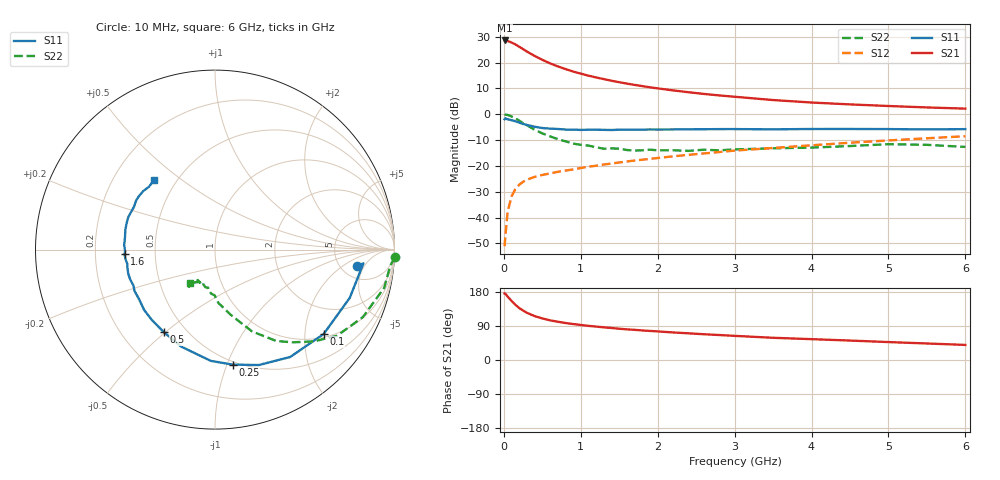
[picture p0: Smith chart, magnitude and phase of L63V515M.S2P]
!  INFINEON TECHNOLOGIES Small Signal Semiconductors
! BFR380L3 , Si-NPN RF-Transistor in TSLP-3-1
!  Vce=3.5 V,  Ic=15 mA
! Common Emitter S-Parameters:  07. March 2005
#  GHz  S  MA  R  50
! f  S11  S21  S12  S22
! GHz  Mag  Ang  Mag  Ang  Mag  Ang  Mag  Ang
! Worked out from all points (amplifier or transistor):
!   36 points, 10 MHz to 6 GHz, reference 50 ohm
!   highest |S21| = 28.5 dB at 10 MHz (marker M1)
!   |S21| within 3 dB of that: start of sweep to 230.8 MHz
!   unconditionally stable (mu >= 1): 2.173 GHz to 4.738 GHz
!   at 250 MHz: K = 0.30, MSG = 25.7 dB, |S12| = -26.1 dB
!   at 1.4 GHz: K = 0.91, MSG = 16.0 dB, |S12| = -19.1 dB
!   at 6 GHz: K = 0.97, MSG = 5.3 dB, |S12| = -8.5 dB
!   S11 on the Smith chart (normalised r, x): 10 MHz: 7.18, -3.53; 100 MHz: 1.10, -2.50; 250 MHz: 0.47, -1.05; 500 MHz: 0.38, -0.49; 1.6 GHz: 0.33, -0.02; 6 GHz: 0.38, +0.40
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0.01  0.7988 -6.4  26.75 175.5  0.0028 73.9  1.003 -2.5
0.02  0.8306 -5.3  26.64 174.9  0.0044 88.3  0.9806 -5.2
0.05  0.7975 -19.7  26.06 167.3  0.0132 83.5  0.9665 -12.7
0.1  0.7666 -37.8  24.4 155.9  0.0256 73.0  0.9059 -24.5
0.15  0.7304 -55.0  22.42 145.6  0.0357 65.7  0.8325 -35.2
0.2  0.688 -69.2  20.2 137.1  0.0431 61.1  0.7525 -42.8
0.25  0.6485 -81.2  18.18 130.5  0.0493 56.2  0.6716 -50.3
0.3  0.6203 -92.2  16.32 124.6  0.0541 54.0  0.6123 -56.2
0.4  0.5721 -109.3  13.44 115.8  0.0613 50.5  0.5011 -65.6
0.5  0.5409 -121.8  11.3 109.7  0.0669 49.8  0.4259 -71.1
0.6  0.5266 -132.1  9.646 104.7  0.0714 49.7  0.3731 -76.5
0.7  0.5185 -139.6  8.443 101.0  0.0768 50.7  0.3306 -81.3
0.9  0.5041 -152.7  6.701 94.9  0.0854 52.0  0.2706 -89.2
1.1  0.501 -160.9  5.575 90.1  0.0965 53.8  0.2471 -94.7
1.4  0.495 -170.9  4.44 84.5  0.1111 56.0  0.2179 -101.3
1.6  0.5045 -177.1  3.911 80.9  0.1219 57.2  0.2029 -108.9
2.2  0.507 171.1  2.892 72.7  0.1531 59.8  0.2008 -114.0
2.8  0.5152 161.2  2.312 65.9  0.1853 61.5  0.2 -121.7
3.5  0.5105 152.0  1.881 58.6  0.2224 60.8  0.2192 -122.7
4.5  0.518 145.0  1.549 51.3  0.2809 60.7  0.2424 -124.1
5.5  0.5081 136.5  1.353 43.6  0.3424 58.2  0.2558 -124.8
6  0.5151 131.1  1.283 39.8  0.3754 56.4  0.2329 -126.3
